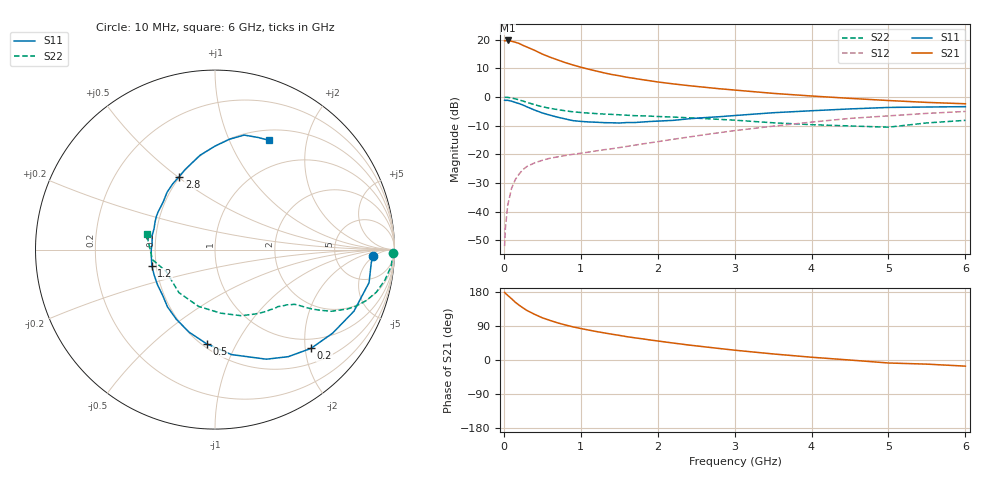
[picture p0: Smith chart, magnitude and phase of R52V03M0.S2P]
! SIEMENS Small Signal Semiconductors
! BFR183
! Si NPN RF Bipolar Junction Transistor in SOT23
! VCE = 2 V  IC = 3 mA
! Common Emitter S-Parameters:  May  1996
# GHz  S  MA  R  50
!  f  S11  S21  S12  S22
! GHz  MAG  ANG  MAG  ANG  MAG  ANG  MAG  ANG
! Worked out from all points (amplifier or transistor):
!   36 points, 10 MHz to 6 GHz, reference 50 ohm
!   highest |S21| = 19.7 dB at 50 MHz (marker M1)
!   |S21| within 3 dB of that: start of sweep to 361 MHz
!   unconditionally stable (mu >= 1): 1.243 GHz to 2.808 GHz
!   at 250 MHz: K = 0.30, MSG = 21.6 dB, |S12| = -25.3 dB
!   at 1.4 GHz: K = 1.05, MAG = 11.6 dB, |S12| = -18.1 dB
!   at 6 GHz: K = 0.90, MSG = 1.3 dB, |S12| = -5.0 dB
!   lowest NFmin = 1.10 dB at 450 MHz
!   S11 on the Smith chart (normalised r, x): 10 MHz: 14, -5; 200 MHz: 0.79, -2.12; 500 MHz: 0.53, -0.77; 1.2 GHz: 0.47, -0.10; 2.8 GHz: 0.50, +0.51; 6 GHz: 0.63, +1.42
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0.01  0.8801 -2.5  9.558 178.5  0.0025 86.1  0.9945 -1.0
0.02  0.8738 -4.8  9.584 176.1  0.0051 88.9  0.9896 -2.1
0.05  0.8779 -12.1  9.707 170.6  0.0129 82.4  0.9862 -5.3
0.1  0.8468 -23.9  9.401 161.7  0.0255 77.8  0.9616 -10.2
0.15  0.8039 -35.4  9.033 152.2  0.0365 71.1  0.9295 -14.8
0.2  0.7676 -45.8  8.586 144.4  0.0456 66.5  0.8896 -18.6
0.3  0.6743 -64.9  7.45 130.8  0.0614 59.1  0.81 -24.1
0.4  0.592 -81.1  6.526 120.5  0.071 53.7  0.7343 -27.9
0.5  0.5277 -94.9  5.616 111.4  0.0787 50.7  0.6761 -30.0
0.6  0.4825 -107.3  4.961 104.4  0.0856 48.9  0.6361 -31.4
0.7  0.4443 -118.9  4.439 98.0  0.0904 48.0  0.603 -32.4
0.8  0.4148 -129.6  3.981 92.4  0.0954 47.5  0.5744 -33.2
0.9  0.3869 -139.1  3.619 87.4  0.1004 48.2  0.5521 -33.9
1.1  0.3677 -157.0  3.063 79.1  0.1094 49.1  0.525 -35.7
1.2  0.3634 -165.4  2.845 75.2  0.1148 49.6  0.5141 -36.7
1.6  0.3588 167.1  2.213 61.5  0.1376 52.2  0.4818 -41.0
2.2  0.3914 137.7  1.697 44.8  0.183 54.4  0.447 -50.3
2.8  0.4532 116.1  1.396 30.4  0.2386 52.5  0.4075 -63.2
3.5  0.5323 99.0  1.159 16.0  0.3102 46.5  0.3555 -84.9
4.5  0.6203 82.5  0.948 -0.1  0.424 34.6  0.3129 -130.0
5.5  0.6694 68.9  0.806 -10.9  0.5186 21.1  0.3534 -171.0
6  0.6797 63.6  0.763 -16.2  0.5601 12.5  0.3917 166.9
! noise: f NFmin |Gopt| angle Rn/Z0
0.45  1.1  0.37  35  0.3
0.9  1.15  0.34  85  0.23
1.8  1.9  0.35  160  0.13
